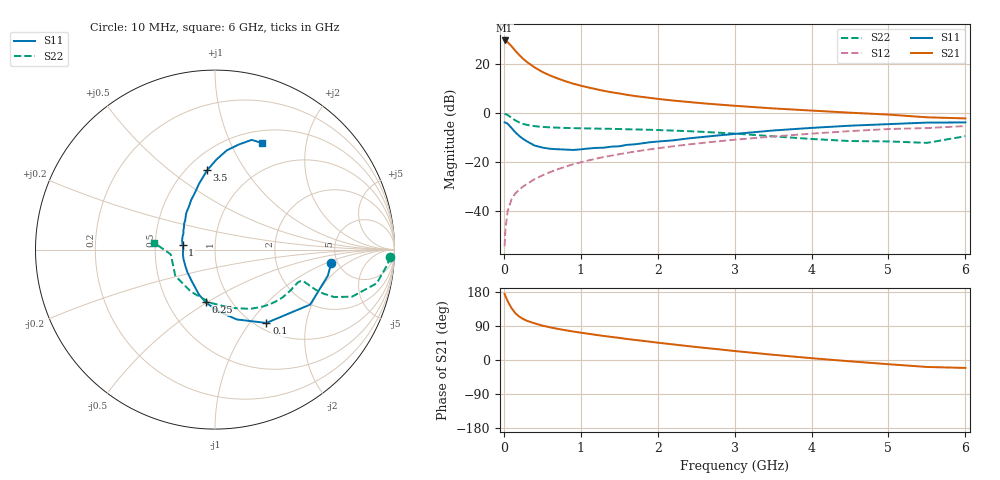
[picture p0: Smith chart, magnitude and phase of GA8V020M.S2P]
! Infineon Technologies  Discrete & RF Semiconductors
! BF775
! Si NPN RF Bipolar Junction Transistor in SOT23
! VCE = 8 V  IC = 20 mA
! Common Emitter S-Parameters:  May  1996
# GHz  S  MA  R  50
!  f  S11  S21  S12  S22
! GHz  MAG  ANG  MAG  ANG  MAG  ANG  MAG  ANG
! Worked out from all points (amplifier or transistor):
!   36 points, 10 MHz to 6 GHz, reference 50 ohm
!   highest |S21| = 29.8 dB at 10 MHz (marker M1)
!   |S21| within 3 dB of that: start of sweep to 116.7 MHz
!   unconditionally stable (mu >= 1): 446.3 MHz to 2.686 GHz
!   at 250 MHz: K = 0.82, MSG = 26.2 dB, |S12| = -30.0 dB
!   at 1.4 GHz: K = 1.09, MAG = 11.1 dB, |S12| = -17.3 dB
!   at 6 GHz: K = 0.90, MSG = 1.6 dB, |S12| = -5.2 dB
!   S11 on the Smith chart (normalised r, x): 10 MHz: 4.44, -1.14; 100 MHz: 1.11, -1.21; 250 MHz: 0.77, -0.49; 1 GHz: 0.69, +0.04; 3.5 GHz: 0.62, +0.69; 6 GHz: 0.65, +1.32
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0.01  0.6522 -6.5  30.97 174.2  0.0019 85.2  0.978 -2.3
0.02  0.6454 -13.0  30.41 169.2  0.0041 83.0  0.9633 -5.1
0.05  0.6125 -30.0  28.56 155.2  0.01 77.0  0.9204 -11.8
0.1  0.4988 -55.0  23.59 136.7  0.0173 68.7  0.8067 -19.0
0.15  0.408 -72.6  18.95 123.5  0.0229 66.2  0.7138 -21.7
0.2  0.3436 -87.4  15.62 114.6  0.0272 65.8  0.6506 -22.1
0.25  0.2983 -99.8  13.06 108.3  0.0316 66.9  0.6067 -21.8
0.3  0.2662 -109.6  11.22 103.5  0.0357 67.9  0.5788 -21.2
0.4  0.2182 -126.5  8.7 96.7  0.0448 68.5  0.5458 -20.3
0.5  0.1987 -141.0  7.031 90.8  0.0534 70.0  0.5257 -19.8
0.6  0.1875 -152.8  5.944 86.3  0.0623 70.3  0.5149 -19.8
0.7  0.1833 -163.0  5.158 82.2  0.0713 70.5  0.5076 -20.3
0.8  0.1807 -171.7  4.529 78.6  0.0805 70.1  0.501 -21.0
1  0.1825 171.5  3.672 72.1  0.099 69.6  0.4926 -22.8
1.1  0.1899 165.0  3.371 69.2  0.1084 69.3  0.4892 -24.1
1.3  0.1973 153.1  2.876 63.5  0.127 68.0  0.4819 -26.5
1.6  0.2256 139.6  2.386 55.5  0.1548 65.5  0.4701 -31.0
2.2  0.279 121.5  1.821 41.2  0.2107 60.2  0.4426 -41.3
3.5  0.4439 95.7  1.258 13.8  0.3344 45.9  0.3374 -74.5
4.5  0.5569 83.2  1.028 -3.5  0.4316 33.3  0.27 -119.7
5.5  0.6447 71.5  0.827 -18.4  0.4981 17.8  0.2477 -173.8
6  0.6486 66.1  0.785 -20.9  0.5473 13.5  0.3392 173.8
